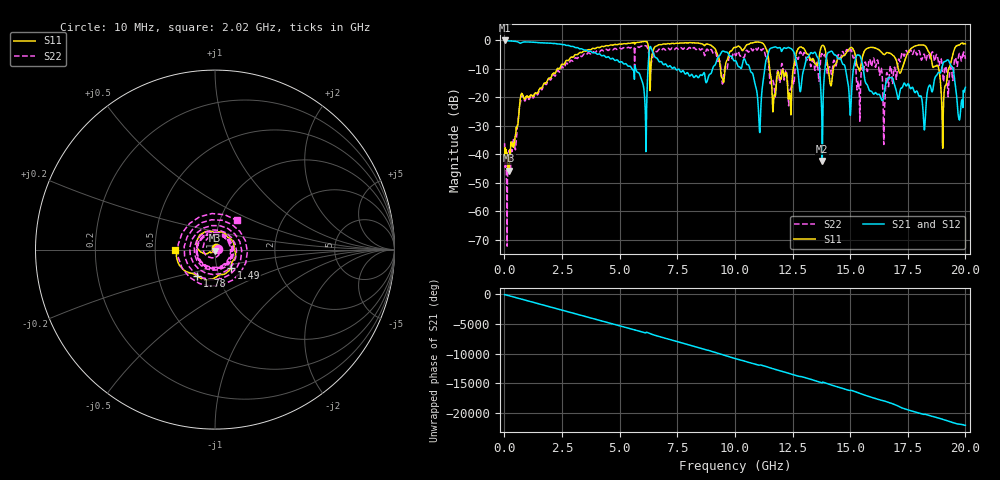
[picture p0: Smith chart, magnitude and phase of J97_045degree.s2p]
!Keysight Technologies,N5222A,MY51421036,A.10.65.16
!Date: Friday, March 31, 2023 15:10:42
!Correction: S11(Full 2 Port(1,2))
!S21(Full 2 Port(1,2))
!S12(Full 2 Port(1,2))
!S22(Full 2 Port(1,2))
!S2P File: Measurements: S11, S21, S12, S22:
# Hz S  dB  R 50
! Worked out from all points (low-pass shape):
!   2000 points, 10 MHz to 20 GHz, reference 50 ohm
!   highest |S21| = -0.06 dB at 10 MHz (marker M1); lowest = -42.3 dB at 13.79 GHz (marker M2)
!   |S21| within 3 dB of the highest: start of sweep to 3.381 GHz; 11.52 GHz to 11.99 GHz (472.7 MHz wide, 4.02 % of centre)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
!   lowest |S11| = -45.7 dB at 180 MHz (marker M3), VSWR 1.01, Z = 49.9 - j0.501 ohm
!   |S11| at or under -10 dB: start of sweep to 2.291 GHz; 11.51 GHz to 12.53 GHz (1.028 GHz wide, 8.55 % of centre); 18.84 GHz to 19.27 GHz (424.3 MHz wide, 2.23 % of centre)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
!   |S22| runs from -72.2 to -1.9 dB; largest |S21 - S12| = 0.009
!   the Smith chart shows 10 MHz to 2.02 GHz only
!   S11 on the Smith chart (normalised r, x): 10 MHz: 1.01, +0.01; 1.49 GHz: 1.17, -0.24; 1.78 GHz: 0.79, -0.24; 2.02 GHz: 0.64, -0.01
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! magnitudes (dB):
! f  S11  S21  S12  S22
! 10 MHz  -40.9  -0.1  -0.1  -36.1
! 180 MHz  -45.7  -0.2  -0.2  -40.3
! 740 MHz  -18.8  -0.9  -0.9  -19.9
! 1.49 GHz  -17.5  -0.8  -0.8  -18.1
! 1.78 GHz  -15.0  -0.9  -0.9  -15.4
! 2.02 GHz  -13.1  -1.0  -1.0  -13.8
! 3.35 GHz  -4.3  -3.0  -3.0  -5.7
! 6.1 GHz  -0.4  -22.3  -22.3  -2.0
! 6.34 GHz  -13.1  -2.2  -2.2  -11.2
! 6.68 GHz  -1.6  -7.1  -7.1  -3.3
! 10.01 GHz  -2.5  -7.1  -7.1  -5.1
! 11.06 GHz  -0.6  -30.7  -30.7  -2.5
! 11.56 GHz  -12.6  -2.8  -2.7  -14.6
! 13.34 GHz  -6.7  -4.4  -4.4  -7.7
! 13.79 GHz  -1.8  -42.3  -42.1  -4.9
! 14.13 GHz  -15.1  -4.1  -4.0  -9.6
! 14.99 GHz  -2.7  -24.5  -24.5  -3.7
! 15.34 GHz  -9.3  -5.2  -5.1  -14.6
! 16.67 GHz  -4.5  -13.1  -13.0  -16.2
! 18.21 GHz  -1.7  -31.0  -30.8  -4.8
! 19.04 GHz  -25.7  -7.9  -7.8  -14.4
! 20 GHz  -1.3  -16.5  -16.4  -6.5
